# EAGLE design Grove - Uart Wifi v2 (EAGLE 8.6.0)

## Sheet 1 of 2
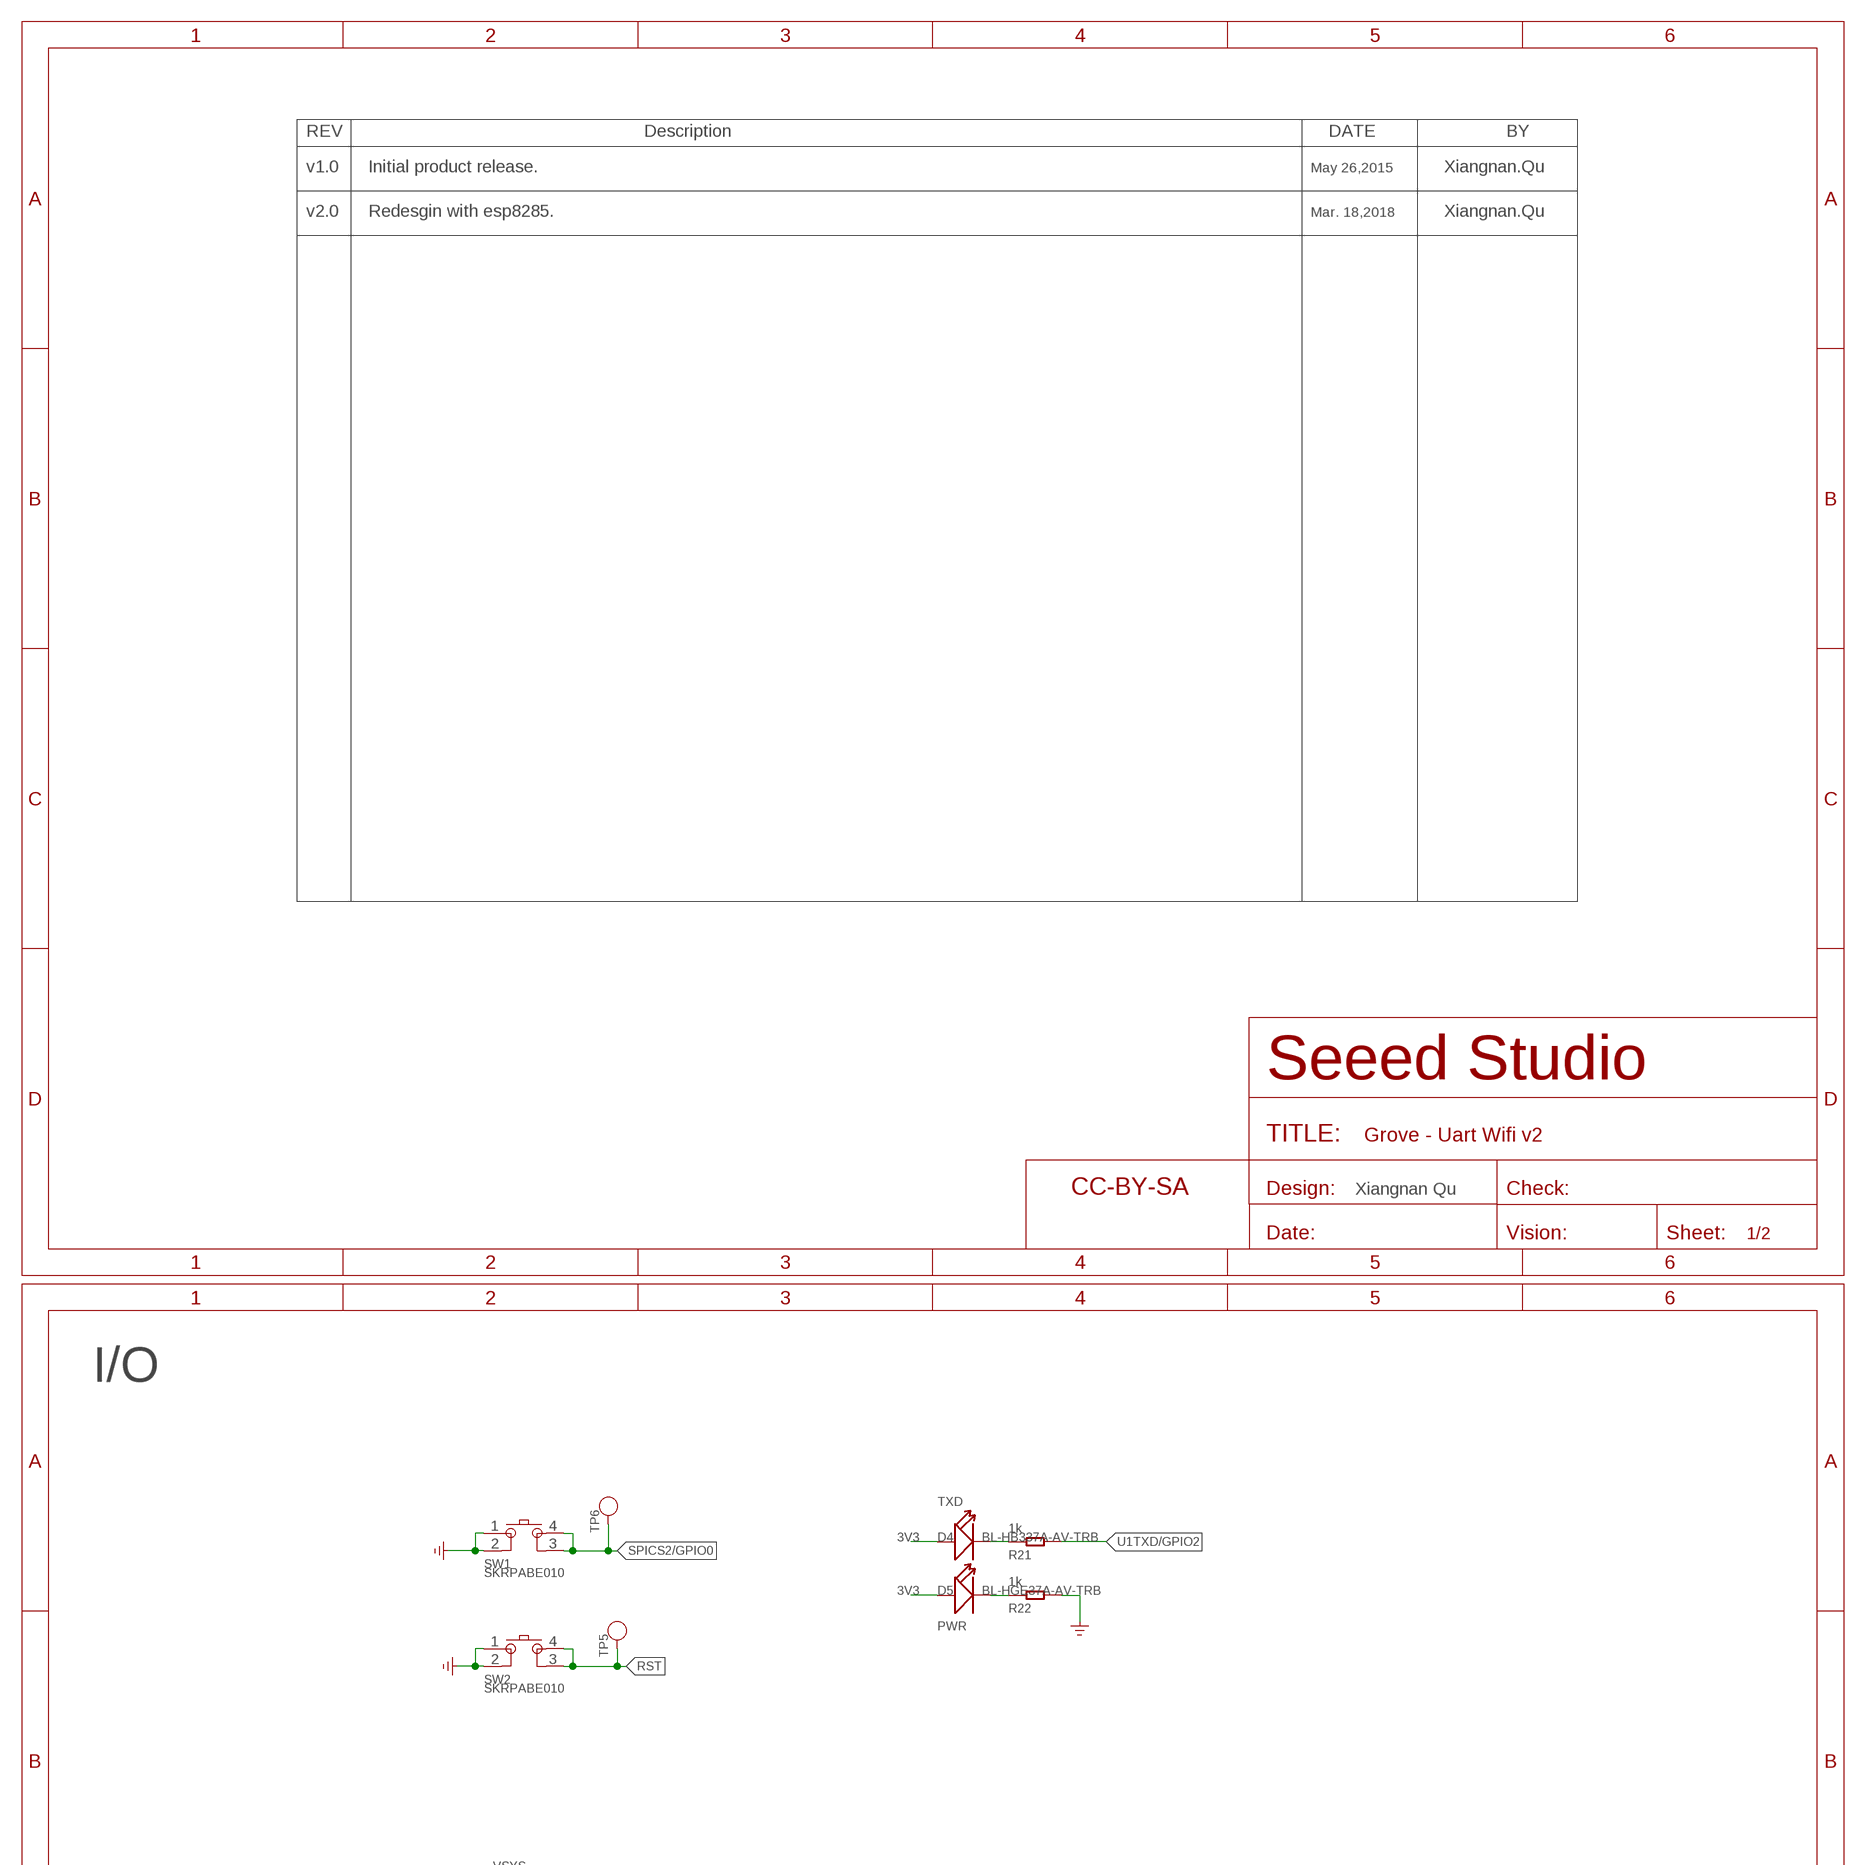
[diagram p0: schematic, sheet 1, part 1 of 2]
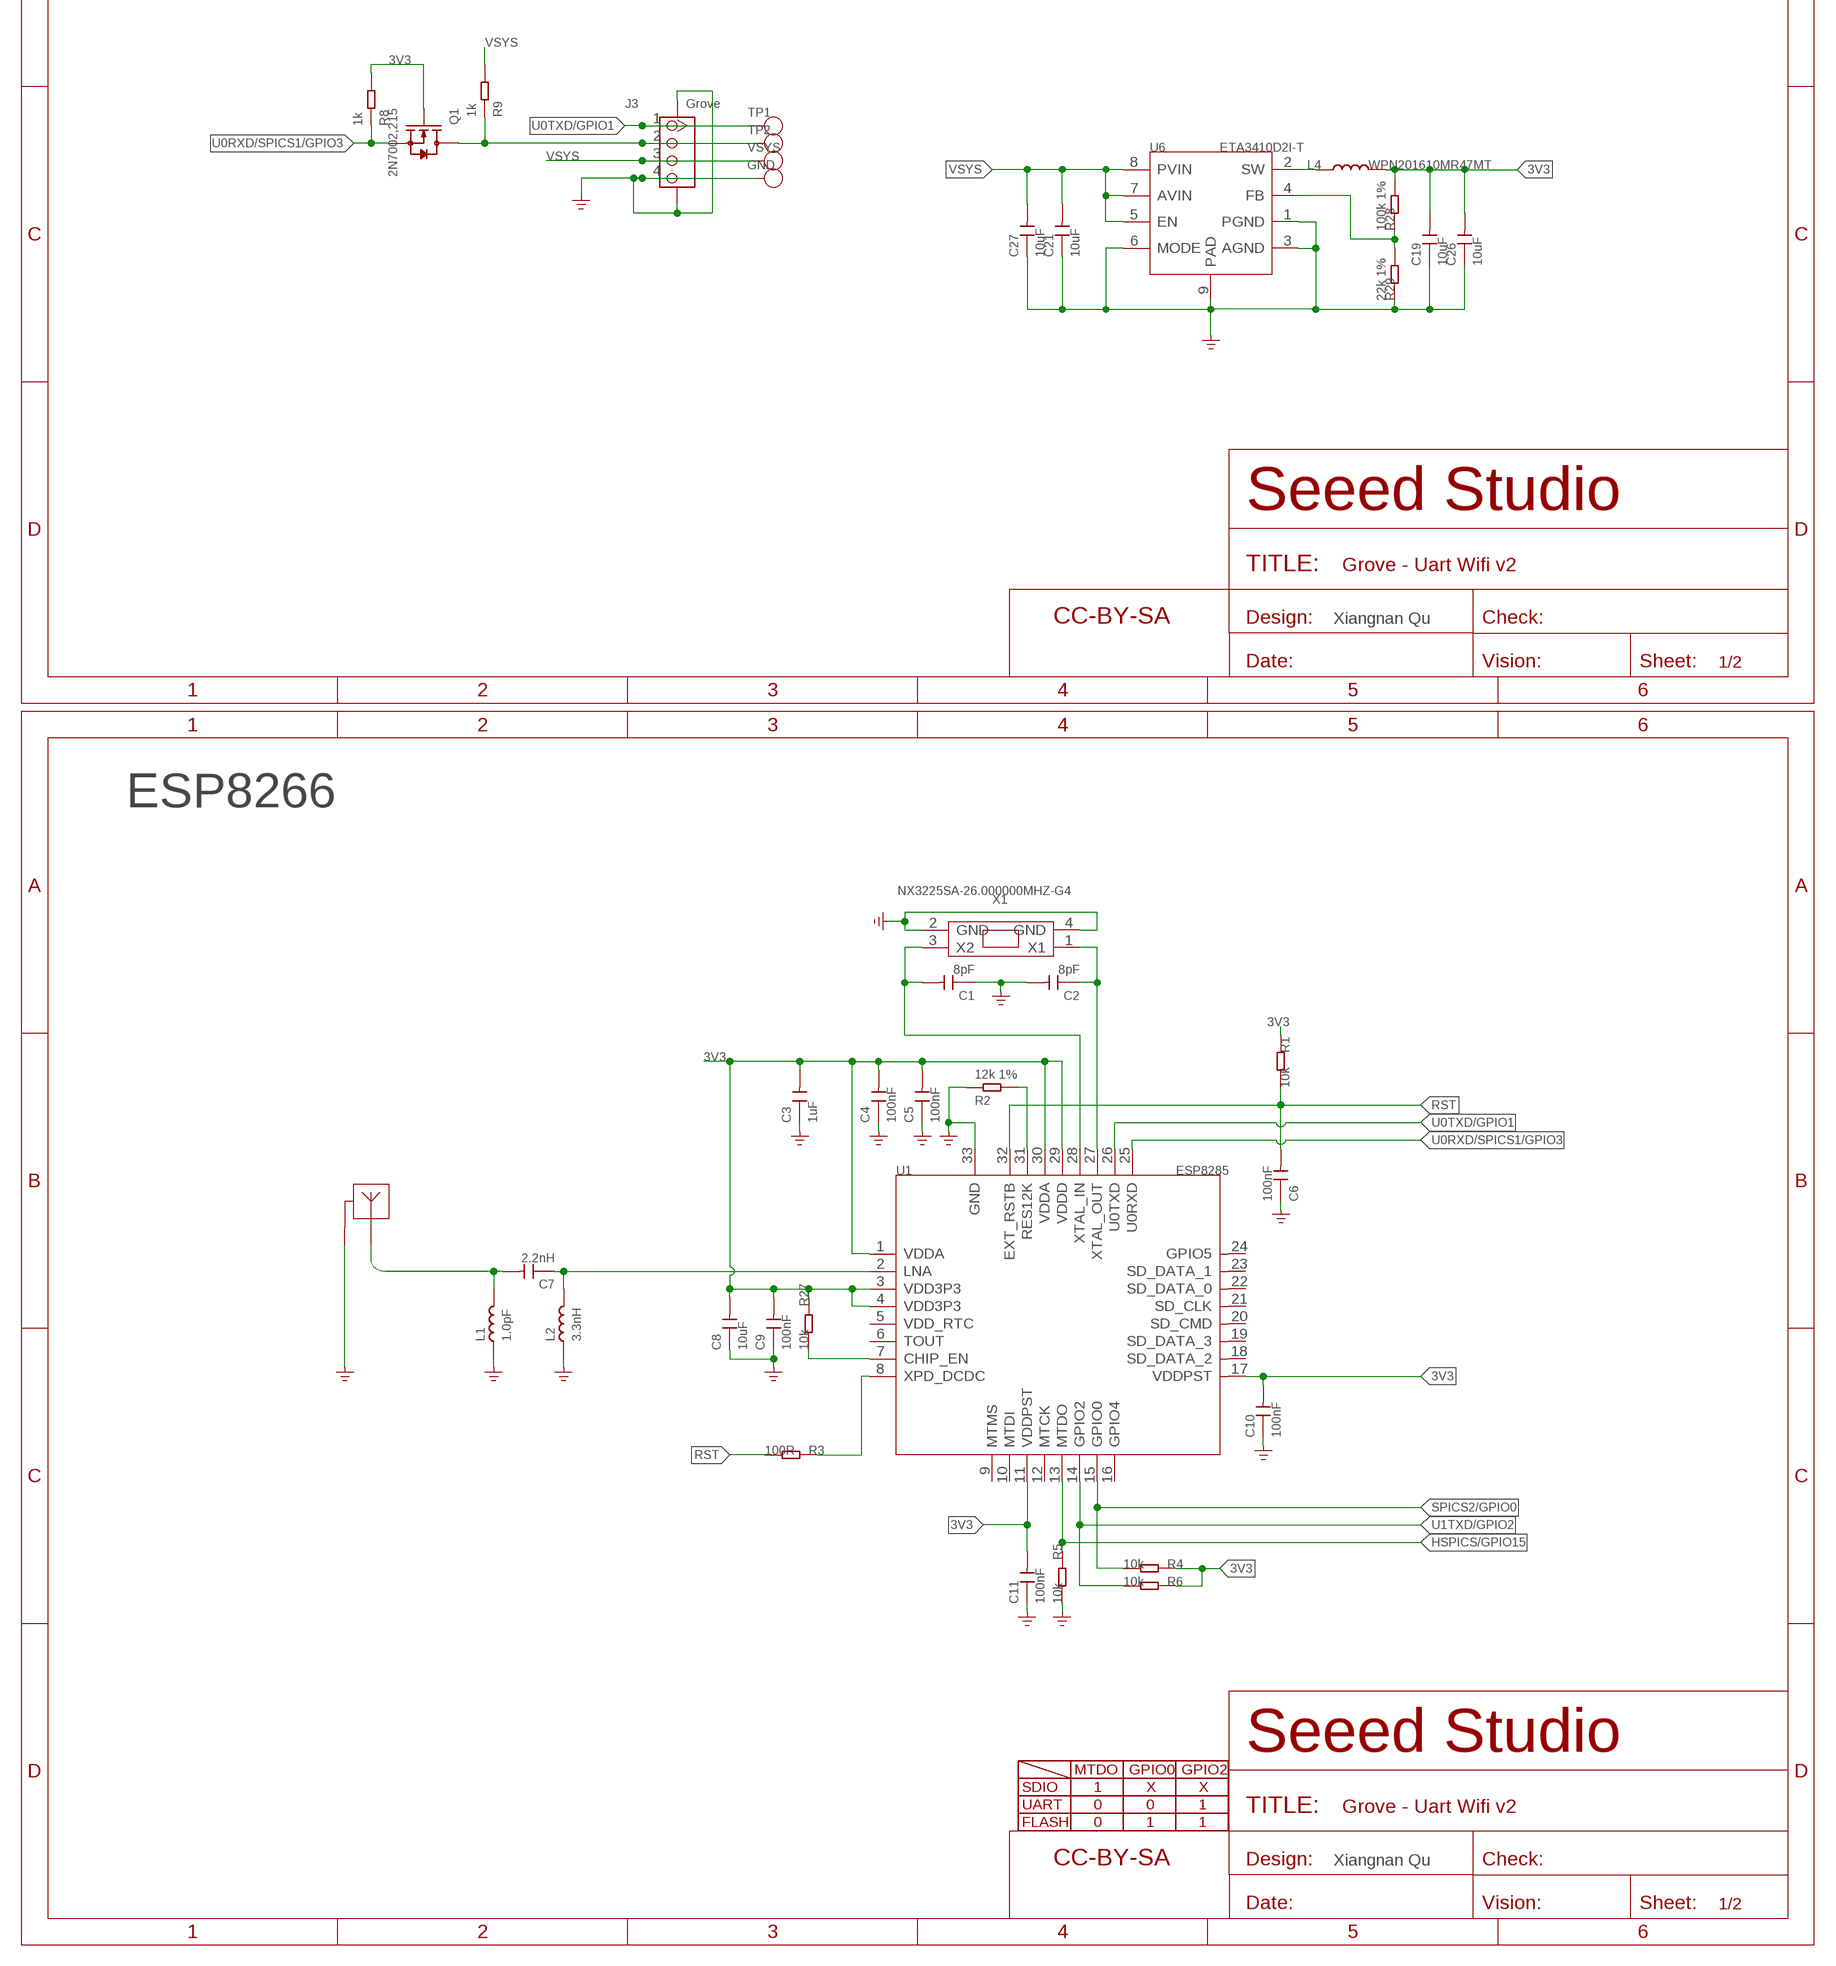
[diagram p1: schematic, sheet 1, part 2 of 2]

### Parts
ANT1  ANTENNA-2.4G-ANTNEW  [2.4G-ANT-NEW]
C1  8pF  CAP-0402  [C0402]
C2  8pF  CAP-0402  [C0402]
C3  1uF  CAP-0402  [C0402]
C4  100nF  CAP-0402  [C0402]
C5  100nF  CAP-0402  [C0402]
C6  100nF  CAP-0402  [C0402]
C7  2.2nH  CAP-0402  [C0402]
C8  10uF  CAP-0603  [C0603]
C9  100nF  CAP-0402  [C0402]
C10  100nF  CAP-0402  [C0402]
C11  100nF  CAP-0402  [C0402]
C19  10uF  CAP-0603  [C0603]
C21  10uF  CAP-0603  [C0603]
C26  10uF  CAP-0603  [C0603]
C27  10uF  CAP-0603  [C0603]
D4  BL-HB337A-AV-TRB  LED-0402  [LED-0402]
D5  BL-HGE37A-AV-TRB  LED-0402  [LED-0402]
FR1  SEEEDSTUDIO-OPEN-SCH-FRAME  [SEEEDSTUDIO-PCB-FRAME]
FR3  SEEEDSTUDIO-OPEN-SCH-FRAME  [SEEEDSTUDIO-PCB-FRAME]
FR4  SEEEDSTUDIO-OPEN-SCH-FRAME  [SEEEDSTUDIO-PCB-FRAME]
GND  TEST-POINT'4545'  [TP-D45MIL]
J3  Grove  GROVE-CONNECTOR-SMD'DD'  [HW4-SMD-2.0]
L1  1.0pF  INDUCTOR/FERRITE-BEAD'0402'  [L0402]
L2  3.3nH  INDUCTOR/FERRITE-BEAD'0402'  [L0402]
L4  WPN201610MR47MT  L-MPM201610SR33_T  [L201610]
Q1  2N7002,215  MOSFET-N'SOT23'  [SOT-23]
R1  10k  RES-0402  [R0402]
R2  12k 1%  RES-0402  [R0402]
R3  100R  RES-0402  [R0402]
R4  10k  RES-0402  [R0402]
R5  10k  RES-0402  [R0402]
R6  10k  RES-0402  [R0402]
R8  1k  RES-0402  [R0402]
R9  1k  RES-0402  [R0402]
R21  1k  RES-0402  [R0402]
R22  1k  RES-0402  [R0402]
R27  10k  RES-0402  [R0402]
R28  100k 1%  RES-0402  [R0402]
R29  22k 1%  RES-0402  [R0402]
SW1  SKRPABE010  BUTTON-4P+  [BUTTON4P-SMD-4.5X3.2X2.5MM]
SW2  SKRPABE010  BUTTON-4P+  [BUTTON4P-SMD-4.5X3.2X2.5MM]
TP1  TEST-POINT'4545'  [TP-D45MIL]
TP2  TEST-POINT'4545'  [TP-D45MIL]
TP5  TEST-POINT'4545'  [TP-D45MIL]
TP6  TEST-POINT'4545'  [TP-D45MIL]
U1  ESP8285  MOUDLE-WIFI-ESP8266EX-ESP8266  [QFN32G-0.5-5X5MM]
U6  ETA3410D2I-T  CONVERTER-ETA3410  [DFN8G-0.5-2X2MM]
VSYS  TEST-POINT'4545'  [TP-D45MIL]
X1  NX3225SA-26.000000MHZ-G4  CRYSTAL-4P'2520'  [X4-SMD-3.2X2.5X0.7MM]

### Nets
3V3: C3.2 C4.2 C5.2 C8.2 C9.2 C10.2 C11.2 C19.2 C26.2 D4.+ D5.+ L4.2 Q1.1(G) R1.1 R4.1 R6.1 R8.2 R27.1 R28.2 U1.1(VDDA) U1.3(VDD3P3) U1.4(VDD3P3) U1.11(VDDPST) U1.17(VDDPST) U1.29(VDDD) U1.30(VDDA)
DSW/GPIO16: R3.1 U1.8(XPD_DCDC)
GND: ANT1.P$1 C1.1 C2.2 C3.1 C4.1 C5.1 C6.1 C8.1 C9.1 C10.1 C11.1 C19.1 C21.1 C26.1 C27.1 GND.T J3.4 J3.SS1 J3.SS2 L1.1 L2.1 R2.2 R5.2 R22.2 R29.1 SW1.1 SW1.2 SW2.1 SW2.2 U1.33(GND) U6.1(PGND) U6.3(AGND) U6.6(MODE) U6.9(PAD) X1.2(GND) X1.4(GND) ; supply symbol labelled GND_POWER
HSPICS/GPIO15: R5.1 U1.13(MTDO)
N$1: R2.1 U1.31(RES12K)
N$2: C1.2 U1.28(XTAL_IN) X1.3(X2)
N$3: C2.1 U1.27(XTAL_OUT) X1.1(X1)
N$5: C7.1 L2.2 U1.2(LNA)
N$6: ANT1.P$2 C7.2 L1.2
N$7: J3.2 Q1.3(D) R9.1 TP2.T
N$8: R27.2 U1.7(CHIP_EN)
N$14: D4.- R21.1
N$22: D5.- R22.1
N$29: L4.1 U6.2(SW)
N$32: R28.1 R29.2 U6.4(FB)
RST: C6.2 R1.2 R3.2 SW2.3 SW2.4 TP5.T U1.32(EXT_RSTB)
SPICS2/GPIO0: R4.2 SW1.3 SW1.4 TP6.T U1.15(GPIO0)
U0RXD/SPICS1/GPIO3: Q1.2(S) R8.1 U1.25(U0RXD)
U0TXD/GPIO1: J3.1 TP1.T U1.26(U0TXD)
U1TXD/GPIO2: R6.2 R21.2 U1.14(GPIO2)
VSYS: C21.2 C27.2 J3.3 R9.2 U6.5(EN) U6.7(AVIN) U6.8(PVIN) VSYS.T
Unconnected: U1.5(VDD_RTC) U1.6(TOUT) U1.9(MTMS) U1.10(MTDI) U1.12(MTCK) U1.16(GPIO4) U1.18(SD_DATA_2) U1.19(SD_DATA_3) U1.20(SD_CMD) U1.21(SD_CLK) U1.22(SD_DATA_0) U1.23(SD_DATA_1) U1.24(GPIO5)

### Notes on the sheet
- v1.0 | Initial product release. | May 26,2015 | Xiangnan.Qu
- v2.0 | Redesgin with esp8285. | Mar. 18,2018 | Xiangnan.Qu
- Xiangnan Qu
- I/O
- TXD
- PWR
- Xiangnan Qu
- ESP8266
- MTDO | GPIO0 | GPIO2
- SDIO | 1 | X | X
- UART | 0 | 0 | 1
- FLASH | 0 | 1 | 1
- Xiangnan Qu

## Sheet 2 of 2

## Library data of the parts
ANT1 = template:ANTENNA-2.4G-ANT
C1-C11 C19 C21 C26 C27 = Discrete-new:CAP: Ceramic Capacitors
D4 D5 = Discrete-new:LED
FR1 FR3 FR4 = moudle-new:SEEEDSTUDIO-OPEN-SCH-FRAME
GND TP1 TP2 TP5 TP6 VSYS = Discrete-new:TEST-POINT; PARTNO: DNP
J3 = Connector-new:GROVE-CONNECTOR-SMD: 4P-SMD-2.0:320110030;4P-SMD-2.0-90D:320110032
L1 L2 = Discrete-new:INDUCTOR/FERRITE-BEAD
L4 = Discrete-new:L
Q1 = Discrete-new:MOSFET-N
R1-R6 R8 R9 R21 R22 R27-R29 = Discrete-new:RES
SW1 SW2 = Discrete-new:BUTTON-4P+
U1 = template:MOUDLE-WIFI-ESP8266EX: ESP8266 is complete and ⾃ into system wi-fi ⺴ collaterals solve ⽅ case, should be able to pick up software ⽤, or through the other ⼀ should ⽤ processing
U6 = IC-new:CONVERTER-ETA3410: 3MHZ 2A High Step-Down Converter in DFN2x2-8L Package
X1 = Discrete-new:CRYSTAL-4P

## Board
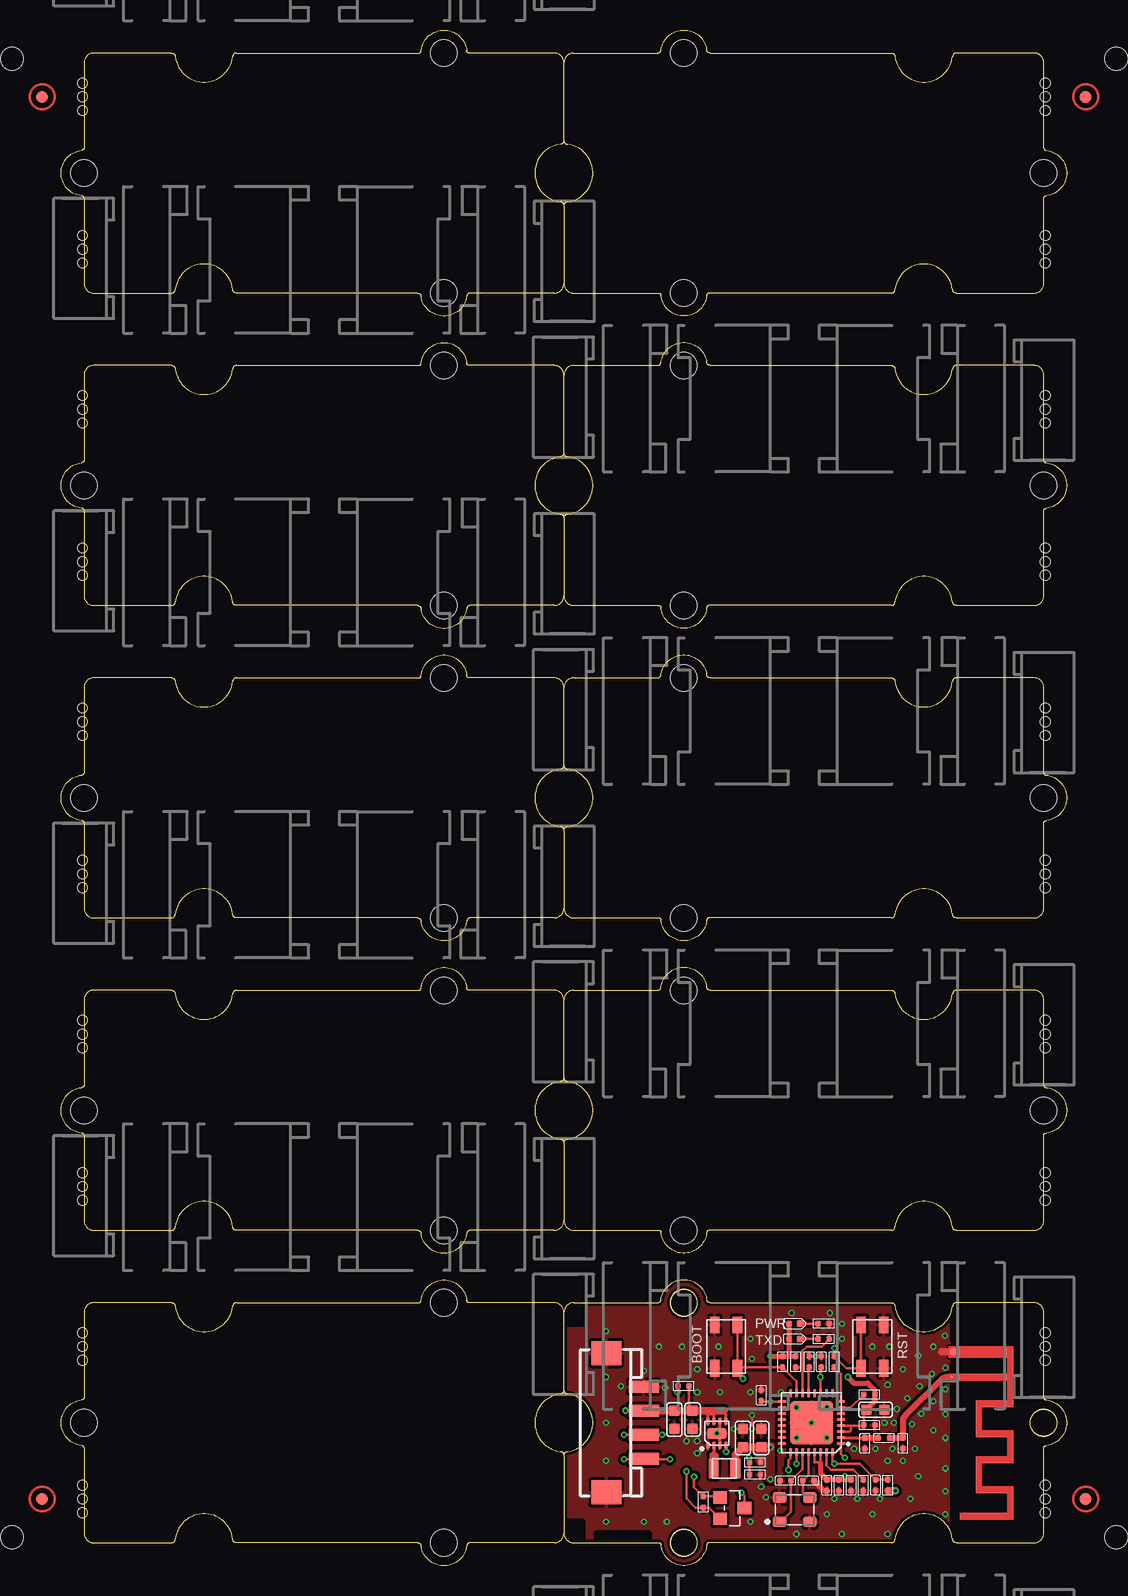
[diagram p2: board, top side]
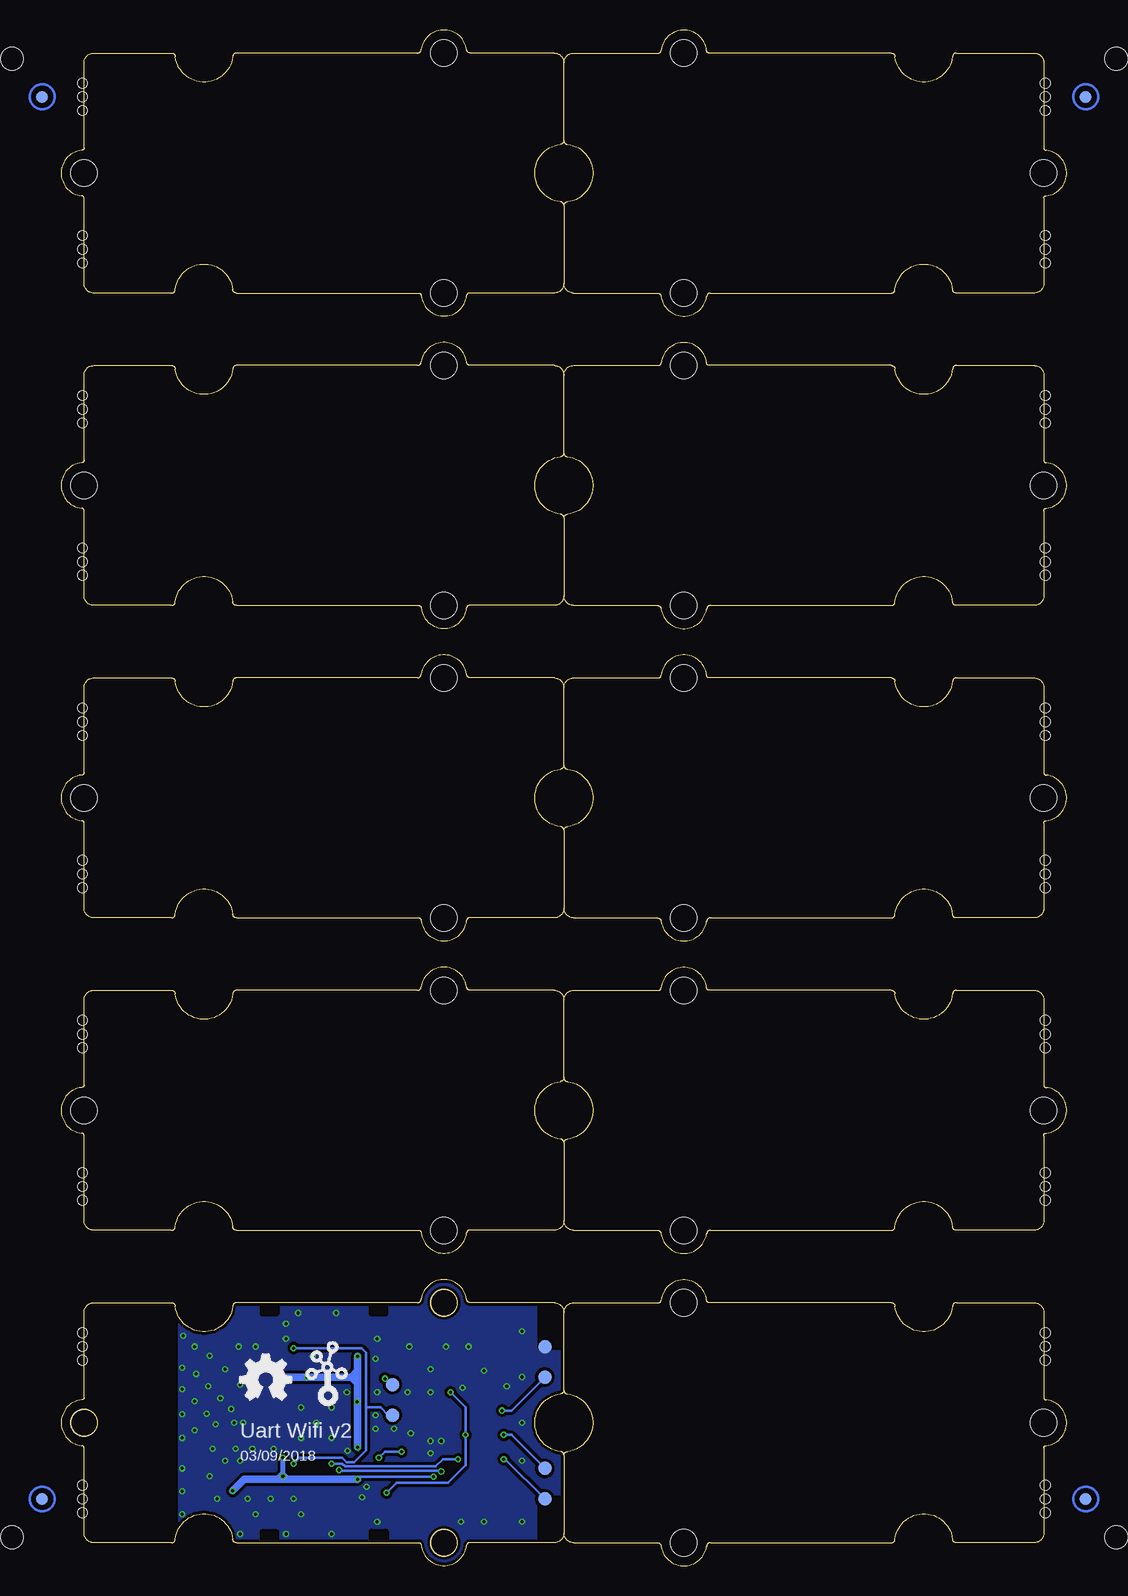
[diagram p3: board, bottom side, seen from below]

Size 83.82 x 127.98 mm. Coordinates in mm from the lower left corner, seen from the top.
Copper layers (1*16): Top 0.035mm / dielectric 1.5mm / Bottom 0.035mm
Design rules "SeeedStudio_2layer_DRU_no_angle_20140221": minimum track width 1mil, minimum drill 10mil, track to track 6mil, track to pad 6mil, pad to pad 6mil, via to via 6mil, smd to smd 0mil, copper to edge 10mil, drill to drill 10mil, minimum pad ring 4mil, minimum via ring 4mil, stop-mask expansion 2mil, vias tented up to drill 25mil, thermal gap 10mil
Holes 0.8 mm at 82.04,4.43 82.04,6.71 82.04,5.57 82.04,17.13 82.04,19.41 82.04,18.27 82.04,30.46 82.04,32.75 82.04,31.61 82.04,43.16 82.04,45.45 82.04,44.31 82.04,56.5 82.04,58.78 82.04,57.64 82.04,69.2 82.04,71.48 82.04,70.34 82.04,82.53 82.04,84.82 82.04,83.68 82.04,95.23 82.04,97.52 82.04,96.38 82.04,108.57 82.04,110.85 82.04,109.71 82.04,121.27 82.04,123.55 82.04,122.41 1.78,6.71 1.78,4.43 1.78,5.57 1.78,19.41 1.78,17.13 1.78,18.27 1.78,32.75 1.78,30.46 1.78,31.61 1.78,45.45 1.78,43.16 1.78,44.31 1.78,58.78 1.78,56.5 1.78,57.64 1.78,71.48 1.78,69.2 1.78,70.34 1.78,84.82 1.78,82.53 1.78,83.68 1.78,97.52 1.78,95.23 1.78,96.38 1.78,110.85 1.78,108.57 1.78,109.71 1.78,123.55 1.78,121.27 1.78,122.41
Holes 1.91 mm at 87.95,125.59 -4.13,125.59 -4.13,2.4 87.95,2.4

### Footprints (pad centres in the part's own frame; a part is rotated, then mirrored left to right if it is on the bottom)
2.4G-ANT-NEW = smd 0.635 x 0.635: P$1 0.45,0.381 | smd 0.254 x 0.254: P$2 2.55,0.254
C0402 = smd 0.5 x 0.5: 1 0,0.463; 2 0,-0.463
C0603 = smd 0.889 x 0.889: 1 0,0.762; 2 0,-0.762
LED-0402 = smd 0.5 x 0.5: + 0.463,0 | smd 0.58 x 0.58: - -0.468,0
TP-D45MIL = smd 1.143 x 1.143: T 0,0
HW4-SMD-2.0 = smd 1 x 2.5: 1 -3,0; 2 -1,0; 3 1,0; 4 3,0 | smd 2 x 2.5: SS1 -5.8,3.123; SS2 5.8,3.123
L0402 = smd 0.5 x 0.5: 1 -0.463,0; 2 0.463,0
L201610 = smd 0.8 x 1.6: 1 -0.9,0; 2 0.9,0
ROUND-MARK-1.0 = smd 1.016 x 1.016: P$1 0,0
SOT-23 = smd 1.143 x 1.016: 1 1.016,-0.889; 2 1.016,0.889; 3 -1.016,0
R0402 = smd 0.5 x 0.5: 1 0,0.463; 2 0,-0.463
BUTTON4P-SMD-4.5X3.2X2.5MM = smd 1.4 x 0.8: 1 -1.8,-0.94; 2 1.8,-0.94; 3 1.8,0.94; 4 -1.8,0.94
QFN32G-0.5-5X5MM = smd 0.7 x 0.25: 1 -2.45,1.75; 2 -2.45,1.25; 3 -2.45,0.75; 4 -2.45,0.25; 5 -2.45,-0.25; 6 -2.45,-0.75; 7 -2.45,-1.25; 8 -2.45,-1.75; 17 2.45,-1.75; 18 2.45,-1.25; 19 2.45,-0.75; 20 2.45,-0.25; 21 2.45,0.25; 22 2.45,0.75; 23 2.45,1.25; 24 2.45,1.75 | smd 0.25 x 0.7: 9 -1.75,-2.45; 10 -1.25,-2.45; 11 -0.75,-2.45; 12 -0.25,-2.45; 13 0.25,-2.45; 14 0.75,-2.45; 15 1.25,-2.45; 16 1.75,-2.45; 25 1.75,2.45; 26 1.25,2.45; 27 0.75,2.45; 28 0.25,2.45; 29 -0.25,2.45; 30 -0.75,2.45; 31 -1.25,2.45; 32 -1.75,2.45 | smd 3.6 x 3.6: 33 0,0
GROVE-TEST-PLATFORM = hole 2.2: -10,-10; -10,10; 20,0
DFN8G-0.5-2X2MM = smd 0.6 x 0.3: 1 -1,0.75; 2 -1,0.25; 3 -1,-0.25; 4 -1,-0.75; 5 1,-0.75; 6 1,-0.25; 7 1,0.25; 8 1,0.75 | smd 0.9 x 1.6: 9 0,0
GROVE-1*2-TEST-PLATFORM-TOP = hole 2.2: 10.635,10; 10.635,-10; -19.365,0
X4-SMD-3.2X2.5X0.7MM = smd 1.143 x 0.889: 1 -1.27,-1.016; 2 1.27,-1.016; 3 1.27,1.016; 4 -1.27,1.016

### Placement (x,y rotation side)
ANT1  73.98,18.27 270 top
C1  62.29,7.1 270 top
C2  60.39,7.1 270 top
C3  63.82,6.71 180 top
C4  65.85,6.71 180 top
C5  64.83,6.71 180 top
C6  67.88,6.73 180 top
C7  68.58,10.65 90 top
C8  67.88,13 270 top
C9  67.37,11.73 270 top
C10  58.37,14.21 0 top
C11  63.37,17 0 top
C19  58.36,10.65 0 top
C21  52.64,12.18 180 top
C26  56.83,10.65 0 top
C27  51.12,12.18 180 top
D4  61.15,18.91 180 top
D5  61.15,20.18 180 top
FR1  not placed on the board
FR3  not placed on the board
FR4  not placed on the board
GND  43.5,18.27 0 bottom
J3  48.58,11.92 90 top
L1  70.17,10.22 90 top
L2  66.99,10.21 90 top
L4  55.31,8.11 0 top
P1  [ROUND-MARK-1.0]  85.41,122.41 180 top
P2  [ROUND-MARK-1.0]  -1.59,122.41 180 top
P3  [ROUND-MARK-1.0]  85.41,5.57 180 top
P4  [ROUND-MARK-1.0]  -1.59,5.57 180 top
P5  [ROUND-MARK-1.0]  85.41,122.41 180 bottom
P6  [ROUND-MARK-1.0]  -1.59,122.41 180 bottom
P7  [ROUND-MARK-1.0]  -1.59,5.57 180 bottom
P8  [ROUND-MARK-1.0]  85.41,5.57 180 bottom
Q1  55.94,4.81 180 top
R1  68.9,6.71 180 top
R2  66.87,6.71 0 top
R3  64.45,17 180 top
R4  60.14,17 0 top
R5  62.36,17 180 top
R6  61.21,17 0 top
R8  53.53,5.32 180 top
R9  51.88,14.97 90 top
R21  63.56,18.91 90 top
R22  63.56,20.19 90 top
R27  67.37,14.27 270 top
R28  57.85,8.62 90 top
R29  57.85,7.6 270 top
SW1  55.44,18.27 270 top
SW2  67.63,18.27 90 top
TP1  43.5,5.57 0 bottom
TP2  43.5,8.11 0 bottom
TP5  56.2,12.56 0 bottom
TP6  56.2,15.1 0 bottom
U1  62.55,11.92 180 top
U2  [GROVE-TEST-PLATFORM]  21.91,90.03 180 top
U3  [GROVE-TEST-PLATFORM]  61.91,90.03 0 top
U4  [GROVE-TEST-PLATFORM]  21.91,63.99 180 top
U5  [GROVE-TEST-PLATFORM]  61.91,63.99 0 top
U6  54.67,11.03 90 top
U7  [GROVE-TEST-PLATFORM]  21.91,37.96 180 top
U8  [GROVE-TEST-PLATFORM]  61.91,37.96 0 top
U9  [GROVE-TEST-PLATFORM]  61.91,11.92 0 top
U10  [GROVE-TEST-PLATFORM]  21.91,11.92 180 top
U11  [GROVE-TEST-PLATFORM]  21.91,116.06 180 top
U12  [GROVE-TEST-PLATFORM]  61.91,116.06 0 top
U$10  [GROVE-1*2-TEST-PLATFORM-TOP]  62.55,11.92 180 top
U$11  [OSHW_FILLX150_NOTEXT]  68.9,13.83 0 bottom
U$12  [GROVE-SILK-SMALL]  63.82,13.19 0 bottom
VSYS  43.5,15.73 0 bottom
X1  61.15,4.68 0 top

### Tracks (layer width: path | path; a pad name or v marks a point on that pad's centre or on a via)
3V3  (via drill 0.25 pad 0.51)
  Top 0.203: U1.11 v63.3,15.73 63.3,16.48 C11.2 | U1.30 63.3,8.62 63.06,8.62 | C5.2 C3.2 | U1.29 62.8,8.75 62.8,8.62 63.06,8.62 | U1.3 65.72,11.17 65.85,11.3 65.85,11.54 | U1.4 65.72,11.67 | 65.72,11.67 65.85,11.67 | 65.85,11.54 65.85,11.67 | 65.72,11.67 65.85,11.54 | U1.17 v59.14,13.67 | v59.14,13.67 58.87,13.67 | 65.85,11.67 65.98,11.67 | 65.98,11.67 66.85,11.67 C9.2 66.91,12.79 C8.2 | U1.1 65,9.34 v65.34,9 | 65.85,11.54 65.98,11.67 | 63.06,8.62 63.18,8.49 | C10.2 58.44,13.67 v59.14,13.67 | Q1.1 54.85,5.78 R8.2 52.77,6.54 v52.77,7.41
  Top 0.406: 65.34,7.18 C4.2 65.64,7.18 v65.34,7.48 | 65.34,7.18 65.09,7.18 | 65.09,7.18 C5.2 63.88,7.16 63.82,7.22 | 63.3,8.62 63.3,7.7 C3.2 | 60.64,17.46 R4.1 59.86,17.45 v59.12,17.45 | 60.64,17.46 R6.1 | D5.+ D4.+ 60.69,17.51 60.64,17.46 | C8.2 67.84,13.72 R27.1 67.84,14.63 67.25,15.22 66.1,15.22 v65.6,15.73 | v65.34,7.48 65.34,7.18 | v65.34,7.48 65.09,7.22 65.09,7.18
  Top 0.61: R1.1 v69.53,6.27 | 56.21,7.72 L4.2 56.21,9.27 C26.2 C19.2 v59.12,9.89
  Bottom 0.203: v59.14,13.67 59.14,13.21 59.12,13.19 | v59.12,7.22 58.93,7.41 v52.77,7.41
  Bottom 0.406: v65.34,9 65.34,7.73 | 65.34,7.73 v65.34,7.48 65.34,7.22 | 65.34,7.73 64.83,7.22 | 65.34,7.73 65.85,7.22
  Bottom 0.61: 59.63,15.73 v63.3,15.73 v65.6,15.73 | 59.63,15.73 59.12,15.73 | 59.12,15.73 59.12,16.24 | 59.12,16.24 v59.12,17.45 | 59.12,15.73 59.12,15.22 | 59.12,15.22 59.12,13.19 v59.12,9.89 | v59.12,7.22 64.83,7.22 65.34,7.22 65.85,7.22 68.58,7.22 v69.53,6.27 | 59.63,15.73 59.12,16.24 | 59.63,15.73 59.12,15.22
  pour Top (no thermals): 58.1,10.27 59.37,10.27 59.37,7.1 59.25,6.97 58.99,6.97 58.87,7.1 58.87,8.11 58.48,8.49 58.1,8.49 57.98,8.62 57.98,10.14
DSW/GPIO16
  Top 0.203: U1.8 65,16.01 R3.1
GND  (via drill 0.25 pad 0.51)
  Top 0.152: v57.6,12.56 v57.6,11.41
  Top 0.203: U6.6 54.92,11.28 U6.9 54.92,10.78 U6.3
  Top 0.406: C3.1 63.6,6.25 C1.1
  Top 0.61: ANT1.P$1 73.4,17.82
  other vias: 67.88,9.76 69.28,9.76 71.18,9.76 69.41,11.92 68.64,11.92 70.55,13.95 73.66,19.16 62.55,11.92 61.28,13.19 63.82,13.19 63.82,10.65 61.28,10.65 54.67,11.03 54.8,18.27 65.09,18.91 65.09,20.18 64.07,21.07 60.9,21.07 67.63,18.27 68.9,15.1 70.17,8.75 70.17,16.37 48.58,3.67 45.4,8.75 45.4,11.92 45.4,15.73 63.82,4.3 64.45,5.57 66.36,5.57 68.26,5.57 67.63,4.3 61.28,2.65 65.09,2.65 68.9,2.65 51.75,18.27 73.72,16.49 72.58,15.99 73.72,12.62 71.57,14.97 73.72,14.72 72.71,13.7 71.69,12.68 70.93,11.79 56.07,11.41 53.02,10.4 52.13,10.4 57.47,3.67 66.1,9.76 68.9,8.75 72.71,11.29 57.47,14.46 54.93,14.46 53.02,14.46 62.87,17.45 49.85,18.27 45.4,3.67 45.4,19.54 53.02,16.37 70.8,5.57 71.44,7.48 72.71,18.27 71.44,17.51 69.03,18.27 60.01,14.46 73.72,4.3 69.66,13.06 73.72,10.65 73.72,8.11 73.72,6.21 58.74,5.7 59.94,9.57 58.36,6.59 53.02,9.38 48.58,16.24 50.36,14.84 46.67,14.97 50.48,3.67 57.6,17.26 57.47,18.91
  pour Bottom (isolate 0.254): 41.59,-0.14 73.98,-0.14 73.98,22.08 73.98,23.99 41.59,23.99
  pour Top (isolate 0.254, rank 6): 41.59,-0.14 73.98,-0.14 73.98,22.08 73.98,23.99 41.59,23.99
  pour Top (no thermals): 73.6,18.65 74.04,18.65 74.04,16.94 73.66,16.94 73.6,16.94
HSPICS/GPIO15
  Top 0.203: U1.13 62.3,16.55 R5.1
N$1
  Top 0.203: U1.31 63.8,8.36 64.17,7.98 66.06,7.98 R2.1
N$2
  Top 0.203: U1.28 62.3,7.54 C1.2 61.85,6.14 62.29,5.7 X1.3
N$3
  Top 0.203: U1.27 61.8,8.06 C2.1 60.83,4.49 60.01,3.67 X1.1
N$5
  Top 0.203: 66.97,10.67 L2.2 | 68.1,10.67 C7.1
  Top 0.254: U1.2 L2.2
  Top 0.508: L2.2 68.1,10.67
N$6
  Top 0.203: 70.14,10.65 L1.2 | ANT1.P$2 73.85,15.72
  Top 0.508: C7.2 70.14,10.65 | 73.85,15.72 arc45 73.4,15.54 70.35,12.49 arc45 70.17,12.04 L1.2
N$7  (via drill 0.25 pad 0.51)
  Top 0.203: 48.85,10.65 48.59,10.91 | v50.1,10.91 48.59,10.91 | 48.59,10.91 J3.2 | R9.1 51.42,14.51 v51.37,14.46 | Q1.3 56.96,5.83 v56.71,6.08 | v46.93,10.91 48.59,10.91
  Bottom 0.203: v51.37,14.46 50.1,13.19 50.1,11.41 v50.1,10.91 50.1,8.37 51.56,6.91 55.88,6.91 v56.71,6.08 | TP2.T 46.29,10.91 v46.93,10.91
N$8
  Top 0.203: R27.2 65.81,13.17 U1.7
N$14
  Top 0.203: R21.1 D4.-
N$22
  Top 0.203: R22.1 61.63,20.19 D5.-
N$29
  Top 0.254: 54.42,9.5 54.42,8.13 L4.1 | U6.2 54.42,9.51 | 54.42,9.51 54.17,9.25 54.17,8.62 54.29,8.49 | 54.42,9.51 54.42,9.5 | 54.42,9.5 54.67,9.25 54.67,8.37 54.55,8.24 54.55,8.87 54.29,9.13 54.29,8.75
N$32  (via drill 0.25 pad 0.51)
  Top 0.203: R29.2 R28.1 57.39,8.96 v57.34,9
  Top 0.254: U6.4 55.42,9.52 v55.44,9.51
  Bottom 0.203: v57.34,9 56.83,9.51 v55.44,9.51
RST  (via drill 0.25 pad 0.51)
  Top 0.203: R1.2 67.9,7.16 C6.2 66.58,8.49 v64.45,8.49 64.3,8.65 U1.32 | SW2.4 SW2.3 | SW2.4 65.45,16.47 R3.2 v64.45,18.14 | 66.61,16.4 SW2.4
  Bottom 0.203: 58.4,13.19 58.4,17.75 58.79,18.14 v64.45,18.14 | 58.4,13.19 58.4,9.65 59.41,8.63 60.03,8.63 60.39,9 63.95,9 v64.45,8.49 | TP5.T 56.58,12.56 57.21,13.19 58.4,13.19
SPICS2/GPIO0  (via drill 0.25 pad 0.51)
  Top 0.203: U1.15 61.3,15.39 R4.2 56.44,16.54 SW1.3 | SW1.3 SW1.4 | v56.83,15.6 56.38,16.06 SW1.3
  Bottom 0.203: TP6.T 56.71,15.6 v56.83,15.6
U0RXD/SPICS1/GPIO3  (via drill 0.25 pad 0.51)
  Top 0.203: v60.64,7.98 60.64,8.81 60.8,8.96 U1.25 | Q1.2 53.99,4.86 R8.1 52.9,4.86 52.13,5.62 v52.13,7.86
  Bottom 0.203: v52.13,7.86 52.11,7.86 52.18,7.92 60.58,7.92 v60.64,7.98
U0TXD/GPIO1  (via drill 0.25 pad 0.51)
  Top 0.203: U1.26 61.3,8.77 v61.28,8.49 | v50.74,8.87 48.63,8.87 | 48.63,8.87 J3.1 | v46.93,8.87 48.63,8.87
  Bottom 0.203: v61.28,8.49 60.39,8.49 60.17,8.28 52.6,8.28 52.01,8.87 v50.74,8.87 | TP1.T 46.8,8.87 v46.93,8.87
U1TXD/GPIO2
  Top 0.203: 61.22,16.56 R6.2 61.75,16.54 61.8,16.49 | R21.2 64.03,18.86 63.44,18.27 62.17,18.27 61.8,17.9 61.8,16.49 | U1.14 61.8,16.49
VSYS  (via drill 0.25 pad 0.51)
  Top 0.203: R9.2 52.34,13.45 | 52.34,13.4 52.34,13.24 C21.2 | 52.34,13.45 52.34,13.4 | 52.34,13.4 52.01,13.06 | 52.34,13.45 52.52,13.27 52.52,13.19 | v47.05,12.94 48.56,12.94 J3.3
  Top 0.254: U6.8 53.92,12.54 | 53.92,12.57 53.92,12.8 53.79,12.94 | U6.5 55.42,12.57 | 55.42,12.57 55.42,12.93 55.18,12.94 | U6.7 54.42,12.55 | 54.42,12.56 54.42,12.93 54.61,12.94 | 53.92,12.54 53.79,12.68 | 53.79,12.68 53.66,12.81 | 53.92,12.54 53.92,12.57 | 53.92,12.57 54.17,12.81 54.42,12.55 | 54.42,12.55 54.42,12.56 | 54.42,12.56 54.67,12.81 | 55.42,12.57 55.18,12.81 | 53.79,12.68 54.42,12.68
  Top 0.61: 55.25,12.94 55.18,12.94 54.61,12.94 53.79,12.94 C21.2 C27.2 51.1,12.92 J3.3
  Bottom 0.203: VSYS.T 46.29,12.94 v47.05,12.94

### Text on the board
tPlace: PWR | TXD | BOOT | RST
bPlace: Uart Wifi v2 | 03/09/2018

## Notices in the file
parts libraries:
moudle-new: This work is licensed under the Creative Commons Attribution 4.0 International License.
To view a copy of this license,visit:
http://creativecommons.org/licenses/by-sa/4.0
moudle-new: CC-BY-SA
